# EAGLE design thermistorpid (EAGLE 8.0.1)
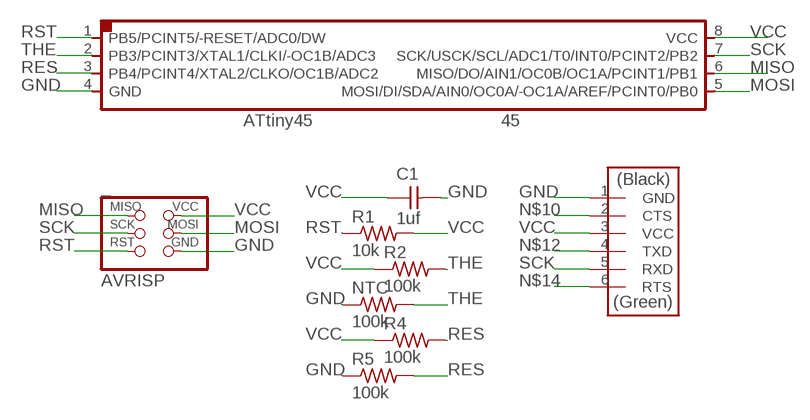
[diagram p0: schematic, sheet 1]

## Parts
45  ATTINY45SI  [SOIC8]
_  AVRISP  AVRISPSMD  [2X03SMD]
__  FTDI-SMD-HEADER  [1X06SMD]
C1  1uf  CAP-UNPOLARIZEDFAB  [C1206FAB]
NTC  100k  RES-US1206FAB  [R1206FAB]
R1  10k  RES-US1206FAB  [R1206FAB]
R2  100k  RES-US1206FAB  [R1206FAB]
R4  100k  RES-US1206FAB  [R1206FAB]
R5  100k  RES-US1206FAB  [R1206FAB]

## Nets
GND: 45.4(GND) _.6(GND) __.1(GND) C1.2 NTC.1 R5.1
MISO: 45.6(MISO/DO/AIN1/OC0B/OC1A/PCINT1/PB1) _.1(MISO)
MOSI: 45.5(MOSI/DI/SDA/AIN0/OC0A/-OC1A/AREF/PCINT0/PB0) _.4(MOSI)
N$10: __.2(CTS)
N$12: __.4(TXD)
N$14: __.6(RTS)
RES: 45.3(PB4/PCINT4/XTAL2/CLKO/OC1B/ADC2) R4.2 R5.2
RST: 45.1(PB5/PCINT5/-RESET/ADC0/DW) _.5(RST) R1.1
SCK: 45.7(SCK/USCK/SCL/ADC1/T0/INT0/PCINT2/PB2) _.3(SCK) __.5(RXD)
THE: 45.2(PB3/PCINT3/XTAL1/CLKI/-OC1B/ADC3) NTC.2 R2.2
VCC: 45.8(VCC) _.2(VCC) __.3(VCC) C1.1 R1.2 R2.1 R4.1

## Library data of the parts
45 = fab:ATTINY45
_ = fab:AVRISP
__ = fab:FTDI-SMD-HEADER
C1 = fab:CAP-UNPOLARIZED
NTC R1 R2 R4 R5 = fab:RES-US: Resistor (US Symbol)

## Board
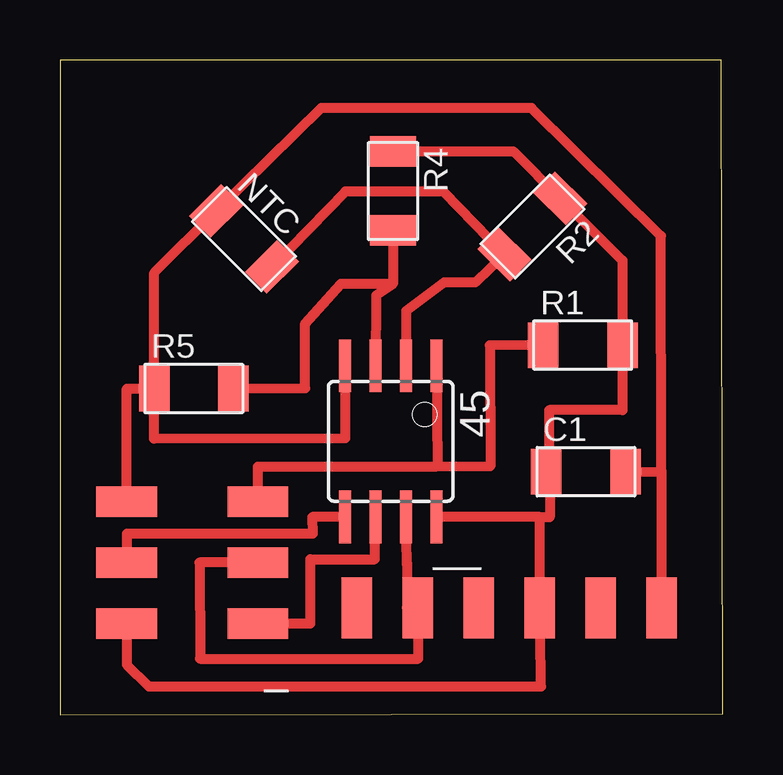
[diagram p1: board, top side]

Size 27.64 x 27.3 mm. Coordinates in mm from the lower left corner, seen from the top.
Outline: 0.02,0 27.64,0.04 27.58,27.28 0,27.3 0.02,0
Copper layers (1*16): Top 0.035mm / dielectric 1.5mm / Bottom 0.035mm
Design rules "default": minimum track width 10mil, minimum drill 24mil, track to track 8mil, track to pad 8mil, pad to pad 8mil, via to via 8mil, smd to smd 8mil, copper to edge 40mil, drill to drill 8mil, minimum pad ring 10mil, minimum via ring 8mil, stop-mask expansion 4mil, vias tented up to drill 0mil, thermal gap 10mil

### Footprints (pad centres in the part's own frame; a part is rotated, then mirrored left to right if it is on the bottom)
SOIC8 = smd 0.5 x 2.2: 1 -1.905,-3.154; 2 -0.645,-3.154; 3 0.625,-3.154; 4 1.895,-3.154; 5 1.905,3.154; 6 0.635,3.154; 7 -0.635,3.154; 8 -1.905,3.154
2X03SMD = smd 2.54 x 1.27: 1 -2.54,2.54; 2 2.92,2.54; 3 -2.54,0; 4 2.92,0; 5 -2.54,-2.54; 6 2.92,-2.54
1X06SMD = smd 2.54 x 1.27: 1 0,6.35; 2 0,3.81; 3 0,1.27; 4 0,-1.27; 5 0,-3.81; 6 0,-6.35
C1206FAB = smd 1.27 x 1.905: 1 -1.651,0; 2 1.651,0
R1206FAB = smd 1.27 x 1.905: 1 -1.651,0; 2 1.651,0

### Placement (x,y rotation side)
45  13.79,11.4 180 top
_  5.71,6.35 180 top
__  18.73,4.46 270 top
C1  21.93,10.13 0 top
NTC  7.67,19.84 315 top
R1  21.8,15.41 0 top
R2  19.7,20.36 225 top
R4  13.89,21.84 270 top
R5  5.58,13.6 0 top

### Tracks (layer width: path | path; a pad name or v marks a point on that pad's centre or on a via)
GND
  Top 0.406: 25.08,10.15 __.1 | 25.08,10.15 25.06,19.96 19.66,25.3 10.89,25.3 NTC.1 3.93,18.43 R5.1 | _.6 2.79,13.6 R5.1 | 45.4 11.89,11.52 3.92,11.5 R5.1 | C1.2 25.08,10.15
MISO
  Top 0.406: _.1 10.44,3.81 10.44,6.48 13.13,6.48 45.6
MOSI
  Top 0.406: 45.5 10.52,8.25 10.54,7.54 2.79,7.54 _.4
RES
  Top 0.406: R5.2 10.22,13.62 10.22,16.32 11.7,17.96 13.88,17.96 | 13.88,17.96 13.18,17.48 45.3 | R4.2 13.88,17.96
RST
  Top 0.406: 15.66,10.34 17.94,10.36 17.92,15.4 R1.1 | 15.66,10.34 8.24,10.34 8.25,9.55 _.5 | 45.1 15.73,10.36 15.66,10.34
SCK
  Top 0.406: 14.46,6.28 14.46,4.46 __.5 14.94,2.34 5.84,2.34 5.82,6.35 _.3 | 14.46,6.28 45.7 | 14.46,6.35 14.46,6.28
THE
  Top 0.406: NTC.2 11.9,21.82 15.98,21.82 R2.2 17.32,18.02 16.02,18.02 14.44,16.84 45.2
VCC
  Top 0.406: R4.1 18.9,23.49 R2.1 23.45,18.94 R1.2 23.45,12.7 20.4,12.7 20.41,10.1 | 20.41,10.1 20.42,8.25 20.02,8.25 | 20.02,8.25 45.8 | 20.02,8.25 __.3 20.04,3.4 20.06,1.18 3.7,1.18 2.79,2.09 _.2 | C1.1 20.41,10.1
